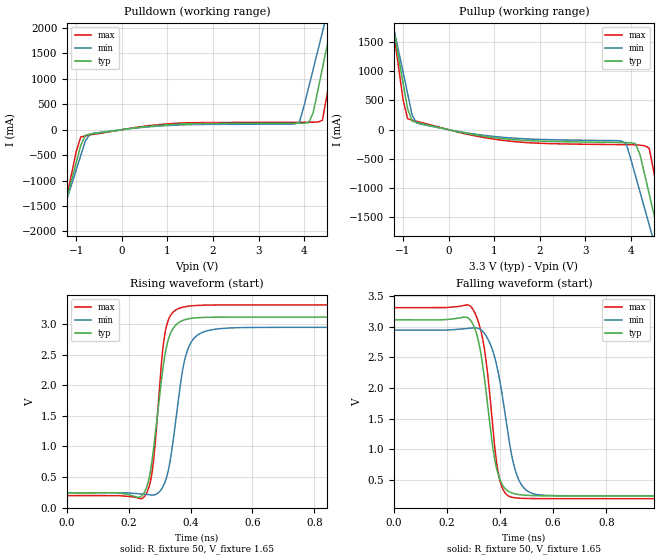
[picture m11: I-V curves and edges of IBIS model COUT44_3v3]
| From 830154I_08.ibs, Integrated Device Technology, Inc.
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[Model] COUT44_3v3
Model_type   Output
Polarity   Non-Inverting
|   typ   min   max
C_comp   2pF   1.5pF   2.5pF
Vmeas = 1.65V
Rref = 50
Cref = 0
Vref = 1.65V
|   typ   min   max
[Voltage range]   3.3V   3.135V   3.465V
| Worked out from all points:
|   slope of the pulldown table from 0 to 0.495 V, typ, clamps not added: 8.59 ohm
|   slope of the pullup table from 0 to 0.495 V, typ, clamps not added: 6.4 ohm
|   rising waveform, R_fixture 50, V_fixture 1.65: 20-80 % time 42ps typ, 46.1ps min, 31.2ps max; typ from 0.243 V to 3.11 V
|   falling waveform, R_fixture 50, V_fixture 1.65: 20-80 % time 52.2ps typ, 64.4ps min, 46.9ps max; typ from 3.11 V to 0.243 V
[Pulldown]
|Voltage   I (typ)   I (min)   I (max)
-3.3V     -8.42A     -7.293A    -10.3A
-1.4V     -2.005A    -1.923A    -2.155A
-1V       -648.7mA   -789.6mA   -430.4mA
-800mV    -111mA     -223.6mA   -120mA
500mV     58.13mA    49.37mA    69.19mA
3.9V      127.6mA    155mA      146.5mA
4.2V      335.4mA    1.189A     148.2mA
4.4V      1.196A     1.91A      182.6mA
4.6V      2.061A     2.634A     1.212A
4.7V      2.495A     2.996A     1.764A
4.8V      2.929A     3.36A      2.317A
6.6V      10.97A     10.07A     12.54A
[Pullup]
|Voltage   I (typ)   I (min)   I (max)
-3.3V     10.95A     9.484A     13.4A
-1.2V     1.684A     1.724A     1.638A
-900mV    358.7mA    616.2mA    188.6mA
-700mV    123.9mA    113.6mA    143.9mA
1.3V      -160.7mA   -137mA     -192.1mA
3.8V      -217.8mA   -194.2mA   -254.9mA
4.1V      -238.7mA   -790.3mA   -258.6mA
4.4V      -1.098A    -1.628A    -317.3mA
4.5V      -1.433A    -1.907A    -715.6mA
4.6V      -1.768A    -2.188A    -1.141A
4.8V      -2.438A    -2.748A    -1.993A
6.6V      -8.477A    -7.801A    -9.667A
[Ramp]
|   typ   min   max
dV/dt_r   1.764/0.043n   1.642/0.046n   1.897/0.031n
dV/dt_f   1.747/0.053n   1.642/0.065n   1.893/0.047n
R_load =   50.0000
[Rising Waveform]
R_fixture = 50
V_fixture = 1.65   |Vcc_typ
V_fixture_min = 1.5675 |Vcc_min
V_fixture_max = 1.7325 |Vcc_max
C_fixture = 0.0p
| Time   typ   min   max
0s        243.1mV    244.6mV    198.5mV
255.3ps   306.4mV    220.9mV    219.9mV
277.8ps   875.3mV    207.1mV    680.4mV
306.3ps   2.119V     309.9mV    2.414V
316.8ps   2.495V     417.5mV    2.845V
334.8ps   2.848V     803.6mV    3.139V
360.4ps   3.019V     1.766V     3.249V
394.9ps   3.086V     2.636V     3.291V
464ps     3.109V     2.9V       3.308V
1.498ns   3.111V     2.945V     3.31V
[Falling Waveform]
R_fixture = 50
V_fixture = 1.65   |Vcc_typ
V_fixture_min = 1.5675 |Vcc_min
V_fixture_max = 1.7325 |Vcc_max
C_fixture = 0.0p
| Time   typ   min   max
0s        3.111V     2.945V     3.31V
298.8ps   3.031V     2.981V     3.275V
319.8ps   2.736V     2.969V     3.055V
339.3ps   2.215V     2.899V     2.679V
373.9ps   991.5mV    2.586V     1.304V
397.9ps   526.8mV    2.143V     520.3mV
433.9ps   312.4mV    1.143V     236.6mV
473ps     264mV      482.7mV    206.3mV
534.5ps   247.3mV    269.1mV    199.8mV
1.498ns   243.1mV    244.6mV    198.5mV
